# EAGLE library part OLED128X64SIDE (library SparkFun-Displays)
Micro OLED TODO: Add description SparkFun Products: Product
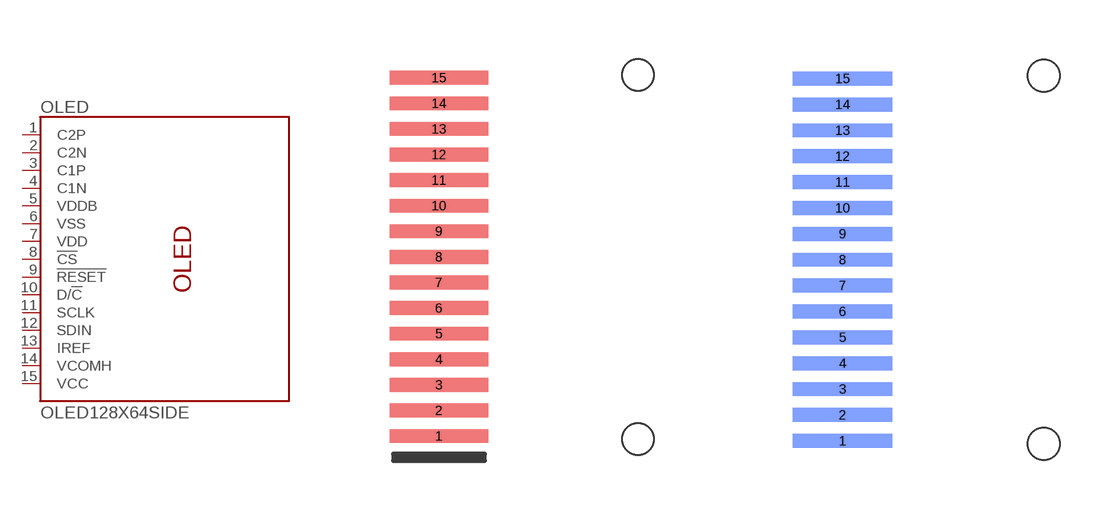
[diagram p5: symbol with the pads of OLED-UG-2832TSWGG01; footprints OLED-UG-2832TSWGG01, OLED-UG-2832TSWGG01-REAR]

Designator prefix OLED

## OLED128X64SIDE (PROD_ID: LCD-13577; VALUE: 32x128 OLED)  [OLED-UG-2832TSWGG01]
1  C2P
2  C2N
3  C1P
4  C1N
5  VDDB
6  VSS
7  VDD
8  !CS!
9  !RESET!
10  D/!C!
11  SCLK
12  SDIN
13  IREF
14  VCOMH
15  VCC

## OLED128X64SIDEREAR-MOUNT (PROD_ID: LCD-13577; VALUE: 32x128 OLED)  [OLED-UG-2832TSWGG01-REAR]
Pads as for OLED-UG-2832TSWGG01

## Footprint OLED-UG-2832TSWGG01 (pad centres in mm)
OLDE display Specifications: Pin count: 30 Pin pitch: 0.7mm Area: Datasheet referenced for footprint: Example device(s): Microview breakout
smd 2.5 x 0.35: 1 0.75,-10.175; 2 0.75,-9.525; 3 0.75,-8.875; 4 0.75,-8.225; 5 0.75,-7.575; 6 0.75,-6.925; 7 0.75,-6.275; 8 0.75,-5.625; 9 0.75,-4.975; 10 0.75,-4.325; 11 0.75,-3.675; 12 0.75,-3.025; 13 0.75,-2.375; 14 0.75,-1.725; 15 0.75,-1.075
hole 0.8 at 5.8,-1
hole 0.8 at 5.8,-10.25

## Footprint OLED-UG-2832TSWGG01-REAR (pad centres in mm)
OLDE display Specifications: Pin count: 30 Pin pitch: 0.7mm Area: Datasheet referenced for footprint: Example device(s): Microview breakout
smd 2.5 x 0.35 bottom: 1 0.75,-10.175; 2 0.75,-9.525; 3 0.75,-8.875; 4 0.75,-8.225; 5 0.75,-7.575; 6 0.75,-6.925; 7 0.75,-6.275; 8 0.75,-5.625; 9 0.75,-4.975; 10 0.75,-4.325; 11 0.75,-3.675; 12 0.75,-3.025; 13 0.75,-2.375; 14 0.75,-1.725; 15 0.75,-1.075
hole 0.8 at 5.8,-1
hole 0.8 at 5.8,-10.25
